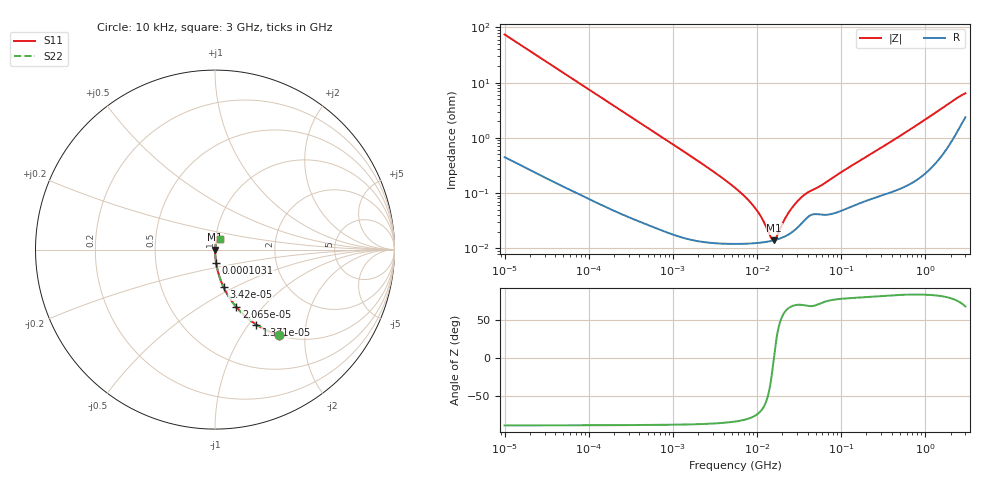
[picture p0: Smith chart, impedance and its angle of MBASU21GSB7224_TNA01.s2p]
! MBASU21GSB7224_TNA01  S-PARAMETER MODEL  ( Standard Model )
! Model Generated by TAIYO YUDEN Corporation (http://www.ty-top.com)
! Version 1.0
! TAIYO YUDEN Control No. 220601
! Copyright(c) 2012 TAIYO YUDEN CO.,LTD. All Rights Reserved.
! Product Description (link to TY-COMPAS)
! https://ds.yuden.co.jp/TYCOMPAS/or/detail?pn=MBASU21GSB7224KTNA01&u=M
! Products Name : Multilayer Ceramic Capacitors
! Characteristics :
!  Capacitance : 0.22 [uF] , Rated Voltage : 50 [V] , TCC : X7R
!  Case Size : 2.0 x 1.25 / 0.079 x 0.049 [mm/inch] , Thickness : 1.25 / 0.049 [mm/inch]
!  (Conditions: Temperature = 25 [degC] , DC Bias Voltage = 0 [V])
! External Node Assignments :
!  1  o---| |---o  2
! GND o---------o GND
! Frequency Range : 10kHz  -  3GHz  [ 401 STEP ]
# MHZ S RI R 50
! Freq[MHz].  S11 Real  S11 Imag  S21 Real  S21 Imag  S12 Real  S12 Imag  S22 Real  S22 Imag
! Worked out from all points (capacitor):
!   401 points, 10 kHz to 3 GHz, reference 50 ohm
!   read as one part in series: C = 213 nF near 10.65 kHz
!   lowest |Z| = 14 mohm at 16 MHz (marker M1)
!   series resonance near 15.88 MHz, so ESL is about 470 pH
!   S11 on the Smith chart (normalised r, x): 10 kHz: 1.01, -1.49; 13.71 kHz: 1.01, -1.09; 20.65 kHz: 1.01, -0.73; 34.2 kHz: 1.00, -0.44; 103.1 kHz: 1.00, -0.15; 3 GHz: 1.05, +0.12
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0.01  0.3591 -0.4768  0.6409 0.4768  0.6409 0.4768  0.3591 -0.4768
0.013707  0.231 -0.4183  0.769 0.4183  0.769 0.4183  0.231 -0.4183
0.020651  0.1181 -0.3192  0.8819 0.3192  0.8819 0.3192  0.1181 -0.3192
0.034199  0.0475 -0.2088  0.9525 0.2088  0.9525 0.2088  0.0475 -0.2088
0.082683  0.00914 -0.0903  0.9909 0.0903  0.9909 0.0903  0.00914 -0.0903
0.103102  0.00609 -0.0728  0.9939 0.0728  0.9939 0.0728  0.00609 -0.0728
0.683653  0.000345 -0.0112  0.9997 0.0112  0.9997 0.0112  0.000345 -0.0112
2.652321  0.000134 -0.00282  0.9999 0.00282  0.9999 0.00282  0.000134 -0.00282
5.477226  0.000121 -0.00124  0.9999 0.00124  0.9999 0.00124  0.000121 -0.00124
7.507384  0.000122 -0.000798  0.9999 0.000798  0.9999 0.000798  0.000122 -0.000798
9.361346  0.000124 -0.000538  0.9999 0.000538  0.9999 0.000538  0.000124 -0.000538
11.67315  0.000128 -0.000304  0.9999 0.000304  0.9999 0.000304  0.000128 -0.000304
14.55585  0.000135 -8.5e-05  0.9999 8.5e-05  0.9999 8.5e-05  0.000135 -8.5e-05
15.99985  0.00014 7.28e-06  0.9999 -7.28e-06  0.9999 -7.28e-06  0.00014 7.28e-06
17.04125  0.000144 6.89e-05  0.9999 -6.89e-05  0.9999 -6.89e-05  0.000144 6.89e-05
21.93027  0.000167 0.000321  0.9998 -0.000321  0.9998 -0.000321  0.000167 0.000321
26.49725  0.000199 0.000522  0.9998 -0.000522  0.9998 -0.000522  0.000199 0.000522
35.19136  0.000301 0.000835  0.9997 -0.000835  0.9997 -0.000835  0.000301 0.000835
45.28751  0.000409 0.00105  0.9996 -0.00105  0.9996 -0.00105  0.000409 0.00105
374.4521  0.00107 0.00812  0.9989 -0.00812  0.9989 -0.00812  0.00107 0.00812
2331.196  0.0142 0.0488  0.9858 -0.0488  0.9858 -0.0488  0.0142 0.0488
3000  0.0264 0.0568  0.9736 -0.0568  0.9736 -0.0568  0.0264 0.0568
